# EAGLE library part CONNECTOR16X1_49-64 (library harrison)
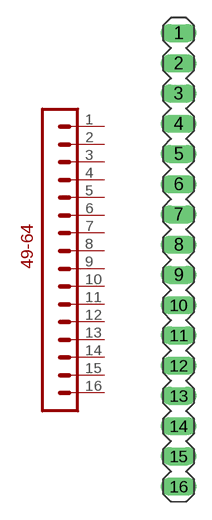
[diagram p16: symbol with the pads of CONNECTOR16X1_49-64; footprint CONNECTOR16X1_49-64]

Designator prefix -

## CONNECTOR16X1_49-64  [CONNECTOR16X1_49-64]
1  P$1  pas
2  P$2  pas
3  P$3  pas
4  P$4  pas
5  P$5  pas
6  P$6  pas
7  P$7  pas
8  P$8  pas
9  P$9  pas
10  P$10  pas
11  P$11  pas
12  P$12  pas
13  P$13  pas
14  P$14  pas
15  P$15  pas
16  P$16  pas

## Footprint CONNECTOR16X1_49-64 (pad centres in mm)
drill 1.016 long: 1 0,12.065; 2 0,9.525; 3 0,6.985; 4 0,4.445; 5 0,1.905; 6 0,-0.635; 7 0,-3.175; 8 0,-5.715; 9 0,-8.255; 10 0,-10.795; 11 0,-13.335; 12 0,-15.875; 13 0,-18.415; 14 0,-20.955; 15 0,-23.495; 16 0,-26.035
